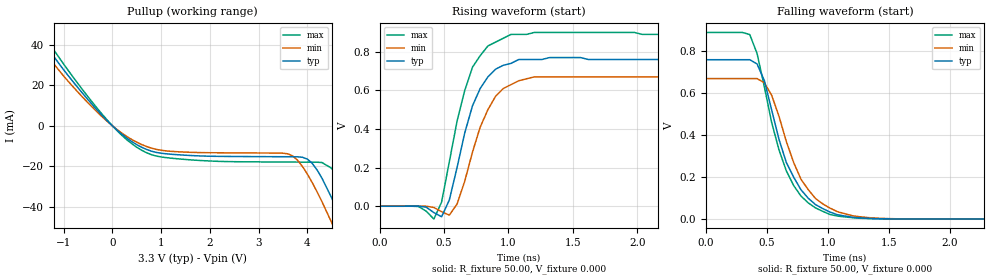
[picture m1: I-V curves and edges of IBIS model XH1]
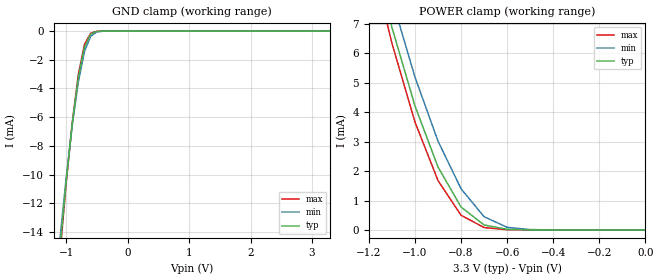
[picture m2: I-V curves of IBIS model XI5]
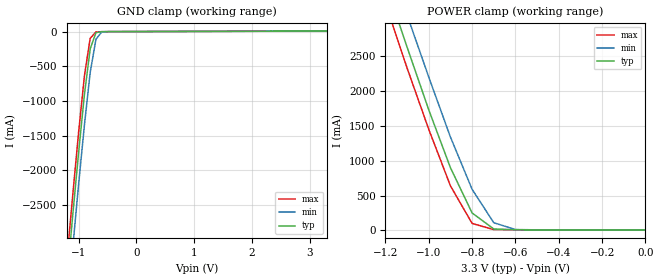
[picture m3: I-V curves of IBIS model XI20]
|   * 9fg108df.ibs * IBIS 2.1 Model for ICS9fg108df
| Rev History
| Rev No.  Description
| 1.0   Initial release with Updated Parasitic Parameters  Sept. 16, 2004
| 1.1   Update CO8, XH1  parasitics. lp
[IBIS Ver]   2.1
[Comment char]  |_char
[File name]   9fg108df.ibs
[Date]   December 18, 2009
[File Rev]   1.1
[Source]   Originated at Integrated Circuit Systems, Inc.
[Disclaimer]
(C) Copyright Integrated Circuit Systems, Inc. 1997
   All rights reserved
ICS hereby grants the user of this 9db109 IBIS model a non-exclusive,
nontransferable license to use this IBIS model under the following terms.
Before using this IBIS model, the user should read this license.
If the user does not accept these terms,  the IBIS model should be
returned to ICS within 30 days.
   The user is granted this license only to use the IBIS model and
is not granted rights to sell, load, rent, lease or license the IBIS
model in whole or in part, or in modified form to anyone other than
user. User may modify the IBIS model to suit its specific
applications but rights to derivative works and such modifications
shall belong to ICS.
   This IBIS model is provided on an "AS IS" basis and ICS makes
absolutely no warranty with respect to the information contained
herein. ICS DISCLAIMS AND CUSTOMER WAIVES ALL WARRANTIES, EXPRESS
OR IMPLIED, INCLUDING WARRANTIES OF MERCHANTABILITY OR FITNESS FOR
A PARTICULAR PURPOSE. The entire risk as to quality and performance
is with the Customer. ACCORDINGLY, IN NO EVENT SHALL THE COMPANY BE
LIABLE FOR ANY DAMAGES, WHETHER IN CONTRACT OR TORT,INCLUDING ANY
LOST PROFITS OR OTHER INCIDENTAL, CONSEQUENTIAL, EXEMPLARY, OR
PUNITIVE DAMAGES ARISING OUT OF THE USE OR APPLICATION OF THE IBIS
model provided in this package. Further, ICS reserves the right to
make changes without notice to any product herein to improve
reliability, function, or design. ICS does not convey any license
under patent rights or any other intellectual property rights,
including those of third parties.
   ICS is not obligated to provide maintenance or support
for the licensed IBIS model.
|   COMPONENT: ICS9fg108df
|This component provides 6*iref (iref=2.32mA) for DIF_T and DIF_C
|0.7V SRC_CLK output
[Component]   ICS9fg108df
[Manufacturer]  ICS
[Package]
| variable   typ   min   max
R_pkg   81.1m   62.2m   100.0m
L_pkg   6.7nH   4.9nH   8.5nH
C_pkg   0.53pF  0.21pF  0.85pF
[Pin]   signal_name   model_name   R_pin   L_pin   C_pin
1   XIN/CLKIN   XIX
2   X2   XIX
3   VDD   POWER
4   VSS   GND
5   REFOUT   CO8
6   FS2   XI20
7   OE_7   XI26
8   DIF_7   XH1
9   DIF_7#   XH1
10   VDD   POWER
11   DIF_6   XH1
12   DIF_6#   XH1
13   OE_6   CI13
14   VDD   POWER
15   GND   GND
16   OE_5   CI13
17   DIF_5   XH1
18   DIF_5#   XH1
19   VDD   POWER
20   DIF_4   XH1
21   DIF_4#   XH1
22   OE_4   XI22
23   SDATA   XIO3
24   SCLK   XI10
25   DIF_STOP#   XI24
26   SPREAD   XI22
27   SEL14M_25M#   XI23
28   OE_3   XI22
29   DIF_3#   XH1
30   DIF_3   XH1
31   VDD   POWER
32   DIF_2#   XH1
33   DIF_2   XH1
34   OE_2   CI13
35   GND   GND
36   VDD   POWER
37   OE_1   CI13
38   DIF_1#   XH1
39   DIF_1   XH1
40   VDD   POWER
41   DIF_0#   XH1
42   DIF_0   XH1
43   OE_0   XI25
44   FS1   XI20
45   FS0   CI24d
46   IREF   XI5
47   GNDA   GND
48   VDDA   POWER
|*  Either 3.3V or 2.5V
|** All model are simulated with typical corner process
[Diff Pin]   inv_pin   vdiff   tdelay_typ
8   9   NA   NA
11   12   NA   NA
16   17   NA   NA
20   21   NA   NA
30   29   NA   NA
33   32   NA   NA
39   38   NA   NA
42   41   NA   NA
| Models and submodels in the file (14): XH1 (Open_source), XI5 (Input), XI20 (Input), XI22 (Input), XI23 (Input), XI24 (Input), XI25 (Input), XI26 (Input), CO8 (Output), CI13 (Input), XIX (Input), CI24d (Input), XI10 (Input), XIO3 (I/O_open_drain)
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|   Model XH1
[Model]   XH1
Model_type   Open_source
Polarity   Inverting
Vmeas = 0.35V
Cref =   2.00pF
Rref =   83
Vref =   0.0V
C_comp   5.50pF   5.00pF   6.00pF
[Temperature Range]   25.00   70.00   0.000
[Voltage Range]   3.30V   3.00V   3.70V
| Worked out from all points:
|   slope of the pullup table from 0 to 0.495 V, typ, clamps not added: 53.7 ohm
|   rising waveform, R_fixture 50.00, V_fixture 0.000: 20-80 % time 196ps typ, 209ps min, 191ps max; typ from 0 V to 0.76 V
|   falling waveform, R_fixture 50.00, V_fixture 0.000: 20-80 % time 266ps typ, 276ps min, 255ps max; typ from 0.76 V to 0 V
[Pullup]
| voltage   I(typ)   I(min)   I(max)
-3.3V     120mA      110mA      120mA
-1.9V     57.97mA    52.49mA    62.98mA
-1.5V     43.73mA    39.31mA    47.78mA
-100mV    2.37mA     2.07mA     2.66mA
700mV     -11.65mA   -10.21mA   -13.27mA
3.6V      -15.27mA   -13.83mA   -17.88mA
4V        -16.4mA    -23.77mA   -17.93mA
4.3V      -25.83mA   -37.4mA    -18.11mA
4.5V      -35.53mA   -47.74mA   -20.97mA
4.7V      -46.5mA    -58.63mA   -28.65mA
5.1V      -70.24mA   -81.19mA   -50.61mA
6.6V      -160mA     -170mA     -150mA
[Ramp]
| variable   typ   min   max
dV/dt_r   0.46/0.20n   0.40/0.21n   0.53/0.19n
dV/dt_f   0.45/0.26n   0.40/0.27n   0.53/0.25n
R_load = 50.00
[Rising Waveform]
R_fixture = 50.00
V_fixture = 0.000
V_fixture_min = 0.000
V_fixture_max = 0.000
| time   V(typ)   V(min)   V(max)
0s        -370nV     -380nV     -340nV
300ps     550uV      230uV      -1.44mV
420ps     -32.86mV   -6.35mV    -66.34mV
480ps     -54.44mV   -28.27mV   21.55mV
540ps     32.24mV    -46.01mV   230mV
600ps     200mV      10.91mV    440mV
720ps     520mV      280mV      720mV
840ps     670mV      500mV      830mV
1.02ns    740mV      630mV      890mV
3ns       760mV      670mV      890mV
[Falling Waveform]
R_fixture = 50.00
V_fixture = 0.000
V_fixture_min = 0.000
V_fixture_max = 0.000
| time   V(typ)   V(min)   V(max)
0s        760mV      670mV      890mV
360ps     760mV      670mV      880mV
420ps     740mV      670mV      790mV
480ps     660mV      650mV      630mV
540ps     520mV      590mV      460mV
660ps     270mV      370mV      230mV
780ps     140mV      190mV      110mV
900ps     68.75mV    97.98mV    52.94mV
1.38ns    2.27mV     4.59mV     1.49mV
3ns       -13.74uV   -37.6uV    -15.05uV
|   Model XI5
[Model]   XI5
Model_type   Input
Polarity   Inverting
Vinl =   0.80V
Vinh =   2.00V
C_comp   5.50pF   5.00pF   6.00pF
[Temperature Range]   25.00   70.00   0.000
[Voltage Range]   3.30V   3.00V   3.70V
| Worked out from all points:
|   GND clamp passes 1 mA (typ) near -0.69 V on its own axis
|   POWER clamp passes 1 mA (typ) near -0.82 V on its own axis
[GND_clamp]
| voltage   I(typ)   I(min)   I(max)
-3.3V     -150mA     -140mA     -150mA
-1.1V     -15.13mA   -14.47mA   -15.58mA
-1V       -10.5mA    -10.27mA   -10.66mA
-900mV    -6.44mA    -6.56mA    -6.36mA
-800mV    -3.2mA     -3.51mA    -2.99mA
-700mV    -1.09mA    -1.4mA     -910uA
-600mV    -220uA     -360uA     -150uA
-500mV    -26.58uA   -59.15uA   -15.29uA
-400mV    -2.29uA    -7.33uA    -1.01uA
3.3V      140pA      140nA      93.85pA
[POWER_clamp]
| voltage   I(typ)   I(min)   I(max)
-3.3V     150mA      140mA      150mA
-1.2V     10.05mA    10.91mA    9.6mA
-1.1V     6.89mA     7.85mA     6.35mA
-1V       4.22mA     5.2mA      3.67mA
-900mV    2.14mA     3.02mA     1.68mA
-800mV    780uA      1.4mA      500uA
-700mV    170uA      450uA      82.21uA
-600mV    22.26uA    89.87uA    8.44uA
-500mV    2.17uA     12.92uA    610nA
0V        140pA      480pA      140pA
|   Model XI20
[Model]   XI20
Model_type   Input
Polarity   Inverting
Enable   Active-High
Vinl =   0.80V
Vinh =   2.00V
C_comp   5.50pF   5.00pF   6.00pF
[Temperature Range]   27.00   70.00   0.000
[Voltage Range]   3.30V   3.00V   3.70V
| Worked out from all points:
|   GND clamp passes 1 mA (typ) near -0.46 V on its own axis
[GND_clamp]
| voltage   I(typ)   I(min)   I(max)
-3.3V     -24.05A    -24.48A    -23.79A
-1.2V     -3.55A     -4.02A     -3.26A
-1.1V     -2.63A     -3.1A      -2.34A
-1V       -1.74A     -2.2A      -1.45A
-900mV    -910mA     -1.35A     -640mA
-800mV    -250mA     -590mA     -98.01mA
-700mV    -15.97mA   -110mA     -5.31mA
-600mV    -2.13mA    -7.05mA    -1.7mA
-500mV    -1.13mA    -1.39mA    -1.09mA
3.3V      6.89mA     6.89mA     6.89mA
[POWER_clamp]
| voltage   I(typ)   I(min)   I(max)
-3.3V     24.05A     24.48A     23.79A
-1.2V     3.55A      4.02A      3.26A
-1.1V     2.63A      3.09A      2.33A
-1V       1.73A      2.2A       1.45A
-900mV    900mA      1.34A      640mA
-800mV    250mA      590mA      100mA
-700mV    20.43mA    110mA      11.13mA
-600mV    8.42mA     12.3mA     9.01mA
0V        6.89mA     6.26mA     7.72mA
